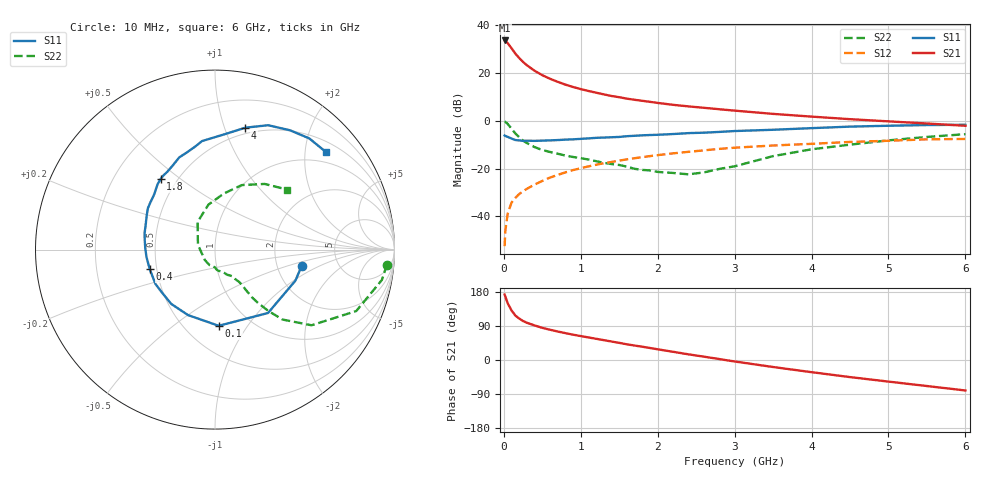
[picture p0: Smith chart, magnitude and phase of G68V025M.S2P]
! SIEMENS Small Signal Semiconductors
! BFG193
! Si NPN RF Bipolar Junction Transistor in SOT223
! VCE = 8 V  IC = 25 mA
! Common Emitter S-Parameters:  August  1996
# GHz  S  MA  R  50
!  f  S11  S21  S12  S22
! GHz  MAG  ANG  MAG  ANG  MAG  ANG  MAG  ANG
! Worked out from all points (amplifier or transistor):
!   36 points, 10 MHz to 6 GHz, reference 50 ohm
!   highest |S21| = 33.5 dB at 10 MHz (marker M1)
!   |S21| within 3 dB of that: start of sweep to 93.86 MHz
!   unconditionally stable (mu >= 1): 662.9 MHz to 2.484 GHz
!   at 250 MHz: K = 0.78, MSG = 27.0 dB, |S12| = -29.5 dB
!   at 1.4 GHz: K = 1.05, MAG = 12.5 dB, |S12| = -17.2 dB
!   at 6 GHz: K = 0.88, MSG = 2.7 dB, |S12| = -7.6 dB
!   S11 on the Smith chart (normalised r, x): 10 MHz: 2.75, -0.66; 100 MHz: 0.72, -0.75; 400 MHz: 0.46, -0.12; 1.8 GHz: 0.41, +0.42; 4 GHz: 0.44, +1.18; 6 GHz: 0.74, +2.48
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0.01  0.4912 -10.7  47.47 172.6  0.0024 83.8  0.9611 -5.0
0.02  0.4803 -21.1  46.4 167.2  0.0051 84.8  0.9452 -10.3
0.05  0.4604 -50.1  41.79 149.7  0.0115 72.4  0.8583 -23.5
0.1  0.425 -87.2  32.6 130.8  0.0195 65.3  0.6833 -38.1
0.15  0.3946 -112.3  25.18 117.2  0.0245 60.8  0.5416 -46.0
0.2  0.3886 -128.8  20.39 109.3  0.0295 61.5  0.4526 -49.0
0.25  0.3803 -141.2  16.88 102.9  0.0335 61.1  0.3834 -51.1
0.3  0.3829 -150.0  14.41 98.2  0.0379 62.1  0.3414 -52.1
0.4  0.3797 -163.4  11.06 91.2  0.0464 62.8  0.2811 -52.6
0.5  0.384 -173.8  8.926 84.8  0.0553 62.8  0.2447 -52.6
0.6  0.3886 178.8  7.525 79.9  0.0649 62.9  0.2225 -53.4
0.7  0.3947 172.6  6.49 75.2  0.0739 61.9  0.2046 -55.1
0.9  0.4088 161.2  5.065 66.8  0.0931 59.4  0.1749 -57.5
1.1  0.4278 152.5  4.182 59.5  0.1112 56.6  0.1548 -64.5
1.4  0.452 140.2  3.285 48.8  0.1376 51.2  0.1245 -75.7
1.8  0.4959 127.7  2.606 35.0  0.1738 43.4  0.0939 -97.3
2.2  0.5273 116.0  2.148 21.7  0.2082 34.6  0.0811 -134.4
3.5  0.6474 84.7  1.39 -18.5  0.3038 4.5  0.1823 122.1
4  0.7 76.0  1.219 -32.1  0.3291 -5.2  0.2531 98.3
4.5  0.7534 66.9  1.078 -45.1  0.3609 -15.3  0.3164 81.0
5.5  0.8122 49.7  0.875 -68.7  0.4087 -38.6  0.4587 52.9
6  0.8237 41.1  0.784 -80.4  0.4164 -52.1  0.5239 39.6
